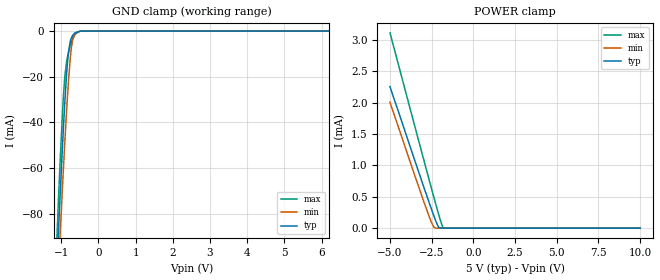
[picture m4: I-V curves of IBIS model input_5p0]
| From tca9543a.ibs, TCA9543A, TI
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|   input_5p0 Model
[Model]   input_5p0
Model_type   Input
Vinl = 1.5
Vinh = 3.5
|   typ   min   max
|   (nom PVT)   (fast PVT)   (slow PVT)
C_comp   1.346e-12   1.280e-12   1.458e-12
[Model spec]
|subparameter
Vinl   1.5   1.35   1.65
Vinh   3.5   3.15   3.85
| Where nom  PVT is Nominal Process, 5V, 27C
|   Fast PVT is Strong Process,  5.5V, -40C
|   Slow PVT is Weak Process,   4.5V, 85C
[Voltage Range]   5   4.5   5.5
|Junction Temperature
[Temperature Range]   27   85   -40
[Power Clamp Reference]   5   4.5   5.5
[GND Clamp Reference]   0   0   0
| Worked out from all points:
|   GND clamp passes 1 mA (typ) near -0.64 V on its own axis
[GND Clamp]
|   Voltage   I(typ)   I(min)   I(max)
-5V       -1.784A    -1.712A    -1.884A
-1.26V    -157mA     -170.4mA   -148.5mA
-1.075V   -87.51mA   -104.3mA   -73.77mA
-1.031V   -71.94mA   -89.36mA   -57.42mA
-936.5mV  -40.67mA   -58.6mA    -27.16mA
-902.5mV  -30.6mA    -48.19mA   -19.68mA
-825mV    -12.36mA   -26.58mA   -10.79mA
-732mV    -3.191mA   -7.923mA   -5.081mA
-695mV    -1.951mA   -3.928mA   -3.411mA
-630.5mV  -779.6uA   -927.2uA   -1.389mA
-380mV    -4.663uA   -3.805uA   -4.702uA
10V       0A         0A         0A
[POWER Clamp]
|   Voltage   I(typ)   I(min)   I(max)
-5V       2.258mA    2.008mA    3.114mA
-3.042V   709.9uA    476.2uA    1.157mA
-2.494V   287.8uA    80.47uA    615.1uA
-2.327V   165.6uA    7.108uA    453.1uA
-2.09V    19.61uA    0A         227.7uA
-2.02V    2.924uA    0A         163.7uA
-1.876V   13.67nA    0A         44.66uA
-1.788V   0A         0A         4.123uA
10V       0A         0A         0A
